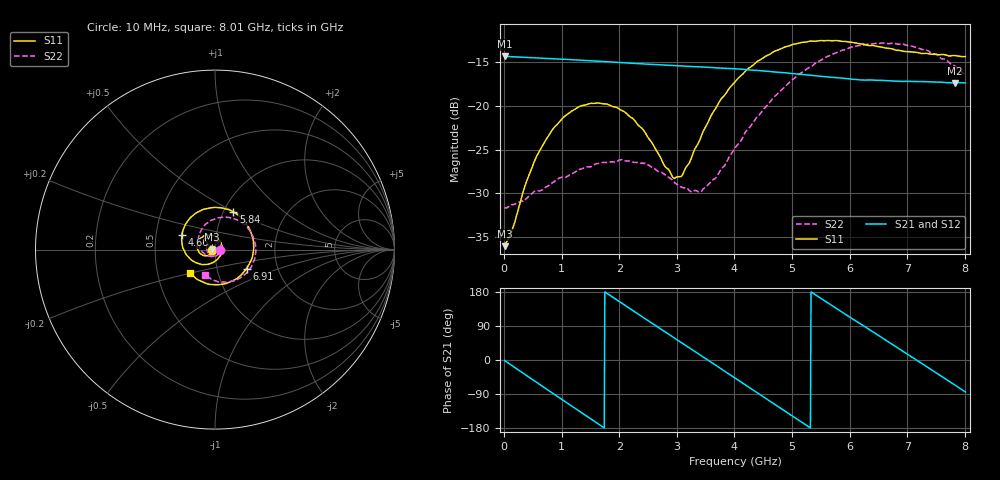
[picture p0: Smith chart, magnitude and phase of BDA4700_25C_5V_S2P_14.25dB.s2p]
!Agilent Technologies,E5071B,MY42404982,A.09.10
!Date: Mon Oct 20 13:33:19 2025
!Data & Calibration Information:
!Freq	S11:SOLT2(ON)	S21:SOLT2(ON)	S12:SOLT2(ON)	S22:SOLT2(ON)
# Hz S RI R 50
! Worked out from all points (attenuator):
!   801 points, 10 MHz to 8.01 GHz, reference 50 ohm
!   highest |S21| = -14.35 dB at 10 MHz (marker M1); lowest = -17.4 dB at 7.83 GHz (marker M2)
!   lowest |S11| = -36.0 dB at 10 MHz (marker M3), VSWR 1.03, Z = 48.4 - j0.123 ohm
!   |S11| at or under -10 dB: start of sweep to end of sweep
!   |S22| runs from -31.7 to -12.8 dB; largest |S21 - S12| = 0.0015
!   S11 on the Smith chart (normalised r, x): 10 MHz: 0.97, -0.00; 4.66 GHz: 0.68, +0.11; 5.84 GHz: 1.11, +0.49; 6.91 GHz: 1.39, -0.31; 8.01 GHz: 0.73, -0.20
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1e7  -0.0158 -0.00127  0.1916 -0.00415  0.1916 -0.00438  0.0263 -0.00103
1.4e8  -0.0171 -0.00957  0.1836 -0.049  0.1837 -0.0491  0.0264 -0.0071
3.8e8  -0.0261 -0.025  0.1448 -0.1208  0.1447 -0.1209  0.0209 -0.0206
6.1e8  -0.0427 -0.0342  0.0832 -0.1673  0.0831 -0.1675  0.0108 -0.0308
1.01e9  -0.0812 -0.0232  -0.0465 -0.1781  -0.0466 -0.1781  -0.0196 -0.0338
1.35e9  -0.0996 0.0111  -0.1379 -0.118  -0.138 -0.1181  -0.0414 -0.0138
1.72e9  -0.0855 0.0565  -0.1785 -0.00879  -0.1785 -0.00885  -0.0438 0.0184
2.08e9  -0.0439 0.0817  -0.1463 0.0975  -0.1463 0.0975  -0.023 0.0428
2.68e9  0.0305 0.0436  0.0121 0.1708  0.0121 0.1709  0.0264 0.0329
2.93e9  0.0387 0.00527  0.0827 0.1479  0.0826 0.1477  0.0348 0.0137
3.08e9  0.0345 -0.0195  0.1177 0.1205  0.1171 0.1209  0.0344 -0.000549
3.43e9  -0.00457 -0.0678  0.1634 0.0308  0.1635 0.0308  0.0156 -0.0287
4.01e9  -0.12 -0.0653  0.1095 -0.1199  0.1095 -0.1197  -0.048 -0.031
4.66e9  -0.1844 0.0802  -0.0614 -0.1432  -0.0611 -0.1437  -0.0926 0.0584
5.35e9  -0.0543 0.2268  -0.1487 0.00589  -0.1489 0.00556  -0.00538 0.1681
5.84e9  0.1025 0.2098  -0.0911 0.1114  -0.0908 0.1114  0.119 0.1671
6.24e9  0.1942 0.1124  -0.0011 0.14  0.000257 0.14  0.201 0.0924
6.68e9  0.2094 -0.0359  0.0944 0.1015  0.0946 0.1016  0.2243 -0.0291
6.91e9  0.1759 -0.1059  0.125 0.0575  0.1251 0.0572  0.2045 -0.0934
7.36e9  0.0519 -0.1911  0.1288 -0.0463  0.129 -0.0465  0.1102 -0.1743
7.83e9  -0.0975 -0.1668  0.0543 -0.1235  0.0541 -0.1238  -0.0166 -0.1672
8.01e9  -0.1406 -0.1289  0.013 -0.1343  0.0132 -0.1345  -0.054 -0.1388
